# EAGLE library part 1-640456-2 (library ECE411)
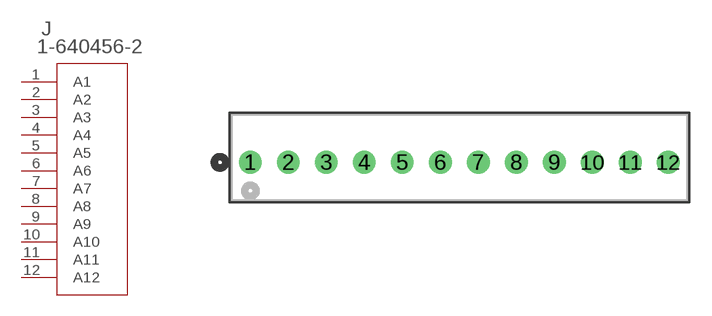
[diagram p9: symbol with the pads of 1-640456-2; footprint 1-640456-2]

Designator prefix J

## 1-640456-2 (MANUFACTURER_PART_NUMBER: 16404562; VENDOR: TE Connectivity)  [1-640456-2]
1  A1  pas
2  A2  pas
3  A3  pas
4  A4  pas
5  A5  pas
6  A6  pas
7  A7  pas
8  A8  pas
9  A9  pas
10  A10  pas
11  A11  pas
12  A12  pas

## Footprint 1-640456-2 (pad centres in mm)
drill 1.016 pad 1.524: 1 -27.94,0; 2 -25.4,0; 3 -22.86,0; 4 -20.32,0; 5 -17.78,0; 6 -15.24,0; 7 -12.7,0; 8 -10.16,0; 9 -7.62,0; 10 -5.08,0; 11 -2.54,0; 12 0,0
